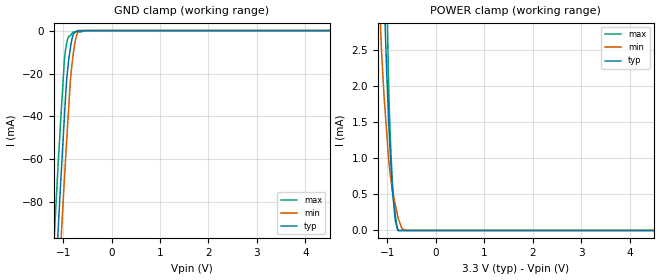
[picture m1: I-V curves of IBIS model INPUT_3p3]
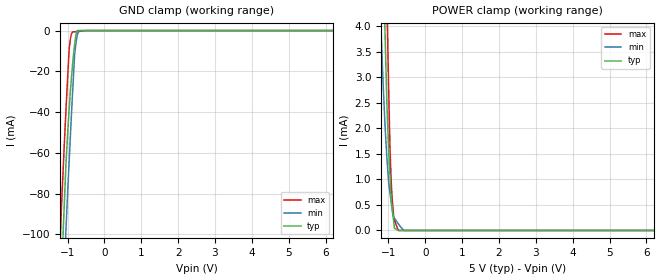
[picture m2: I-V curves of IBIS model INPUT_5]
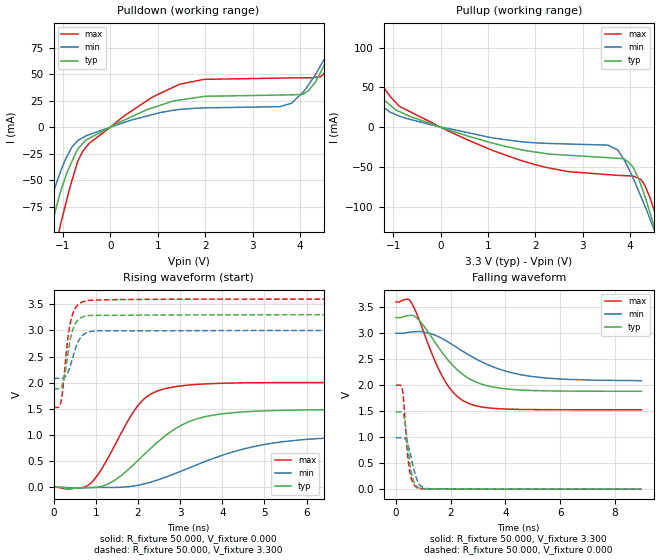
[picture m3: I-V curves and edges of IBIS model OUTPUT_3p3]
|Texas Instruments Incorporated
|14-Bit, Quad Channel, Serial Interface, Multiplying Digital-to-Analog Converter
| Marketing part#   Digital Voltage Range   Package-type   #pins
| DAC8803IDBR   2.7V to 5.5V   SSOP   28
| DAC8803IDBRG4   2.7V to 5.5V   SSOP   28
| DAC8803IDBT   2.7V to 5.5V   SSOP   28
| DAC8803IDBTG4   2.7V to 5.5V   SSOP   28
[IBIS Ver]   3.2
[File name]   dac8803.ibs
|SIMDE Ver   V2.0 - 201002 - RHL4 - Build 372
[Date]   08/20/2010
[File Rev]   1.1
[Source]
| Texas Instruments Incorporated.
| Analog eLab Design Center, HPA
| 12500 TI Blvd
| Dallas, TX -75243
| e-Mail: elab_scm_ibis@list.ti.com
| Model generated from simulations in TISPICE
[Notes]   Revision_History:
|   Rev 1.0: 08/02/2010
|   - Initial version of the model
|   - Model names with a trailing _3p3 contains the model for
|   3V [3 - 3.3 - 3.6]. Model names with trailing _5 contains
|   the model for 5V [4.5 - 5.0 - 5.5] operation.
|   - Model generated from simulations in TISPICE
|   - Model matched to SPICE simulation
|   - While calculating R_pkg, L_pkg and C_pkg ignored values
|   corresponding to power and ground pins
|   - Added package details beside [Package]
|   - C_comp although listed in numerical order of value are
|   obtained from varying PVT conditions. For PVT conditions
|   for each specific value refer the buffer description under
|   respective [Model]. IBIS model user is responsible for using
|   appropriate C_comp to simulate for Signal Integrity.
|   Rev 1.1: 08/20/2010
|   - Re-released after removing INPUT_EN buffers and using INPUT
|   instead
|   - Updated all analog pins as TERM
[Disclaimer]
| This model is designed as an aid for customers of Texas Instruments.
| TI and its licensors and suppliers make no warranties, either expressed
| or implied, with respect to this  model, including the warranties of
| merchantability or fitness for a particular purpose. The model is
| provided solely on an "as is" basis. The entire risk as to its quality
| and performance is with the customer.
[Copyright]
| (C) Copyright 2010 Texas Instruments Incorporated. All rights reserved.
|   DAC8803
[Component]   DAC8803
[Manufacturer]  TI
[Package]  | 28 SSOP - DB package
| variable   typ   min   max
R_pkg   0.03644   0.00363   0.05238
L_pkg   3.09853nH   1.17548nH   4.86282nH
C_pkg   0.73875pF   0.35147pF   1.22787pF
|-------------------------PIN------------------------------------------------
[Pin]  signal_name model_name   R_pin   L_pin   C_pin
1   AGNDA   GND   0.03184   5.81591nH   1.29735pF
2   IOUTA   TERM   0.04659   4.86134nH   1.22696pF
3   VREFA   TERM   0.02815   4.00710nH   1.00527pF
4   RFBA   TERM   0.03031   2.81959nH   0.71201pF
5   MSB   INPUT   0.05211   2.64328nH   0.50891pF
6   _RS   INPUT   0.04857   2.33897nH   0.44307pF
7   VDD   POWER   0.02476   2.03620nH   0.46247pF
8   _CS   INPUT   0.04562   2.25151nH   0.43554pF
9   CLK   INPUT   0.04863   2.34561nH   0.44303pF
10   SDI   INPUT   0.05238   2.65862nH   0.51001pF
11   RFBB   TERM   0.03030   2.82161nH   0.71298pF
12   VREFB   TERM   0.02744   3.75266nH   0.95519pF
13   IOUTB   TERM   0.04608   4.68935nH   1.17882pF
14   AGNDB   GND   0.03363   6.46641nH   1.45119pF
15   AGNDC   GND   0.03286   6.18883nH   1.39946pF
16   IOUTC   TERM   0.04625   4.74353nH   1.19893pF
17   VREFC   TERM   0.02759   3.80912nH   0.95675pF
18   RFBC   TERM   0.03017   2.73838nH   0.68849pF
19   NC   NC   0.00363   1.17548nH   0.37105pF
20   SDO   OUTPUT   0.04717   2.29948nH   0.43486pF
21   _LDAC   INPUT   0.04546   2.24617nH   0.43309pF
22   AGNDF   GND   0.04609   2.26472nH   0.43205pF
23   VSS   NC   0.00371   1.17578nH   0.35147pF
24   DGND   GND   0.02988   2.49325nH   0.54126pF
25   RFBD   TERM   0.03031   2.82053nH   0.71469pF
26   VREFD   TERM   0.02815   4.00814nH   1.00483pF
27   IOUTD   TERM   0.04661   4.86282nH   1.22787pF
28   AGNDD   GND   0.03187   5.81892nH   1.29817pF
|   Model Selectors
[Model Selector]  INPUT
INPUT_3p3  3V digital input
INPUT_5   5V digital input
|NOTES   Model INPUT split into two Models INPUT_3p3 and INPUT_5
|   to accomodate vast voltage range of 2.7V - 5.5V
|   INPUT_3p3 operates in voltage range of 3.0 - 3.3 - 3.6
|   INPUT_5 operates in voltage range of 4.5 - 5.0 - 5.5
|   The max pin frequency for Model INPUT is 20MHz
|   This is referenced with datasheet
[Model Selector]  OUTPUT
OUTPUT_3p3   3V digital output
OUTPUT_5   5V digital output
|NOTES   Model OUTPUT split into two Models OUTPUT_3p3 and OUTPUT_5
|   to accomodate vast voltage range of 2.7V - 5.5V
|   OUTPUT_3p3 operates in voltage range of 3.0 - 3.3 - 3.6
|   OUTPUT_5 operates in voltage range of 4.5 - 5.0 - 5.5
|   The max pin frequency for Model OUTPUT is 12.5MHz
|   This is referenced with datasheet
[Model selector] TERM
TERM_3p3  3.3V nominal termination
TERM_5   5.0V nominal termination
|   Termination - TERM_3p3
[Model] TERM_3p3
Model_type Terminator
C_comp   1.0e-20F  1.0e-20F  1.0e-20F
| variable   typ   min   max
[Voltage Range]   3.30000v  3.00000V  3.60000V
[POWER Clamp Reference]  3.30000v  3.00000V  3.60000V
[GND Clamp Reference]   0.00000V  0.00000V  0.00000V
|Ambient Temperature   25   85   -40
|Junction Temperature
[Temperature Range]   25   85   -40
|   Termination - TERM_5
[Model] TERM_5
Model_type Terminator
C_comp   1.0e-20F  1.0e-20F  1.0e-20F
| variable   typ   min   max
[Voltage Range]   5.00000V  4.50000V  5.50000V
[POWER Clamp Reference]  5.00000V  4.50000V  5.50000V
[GND Clamp Reference]   0.00000V  0.00000V  0.00000V
|Ambient Temperature   25   85   -40
|Junction Temperature
[Temperature Range]   25   85   -40
| Models and submodels in the file (6): INPUT_3p3 (Input), INPUT_5 (Input), OUTPUT_3p3 (Output), OUTPUT_5 (Output), TERM_3p3 (Terminator), TERM_5 (Terminator)
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|   Input INPUT 3 Model
[Model] INPUT_3p3
Model_type Input
| Signals   MSB(5), _RS(6), _LDAC(21)
Vinl = 0.6
Vinh = 2.1
|   typ   min   max
|   (nom PVT)   (Fast PVT)   (slow PVT)
C_comp   7.483e-13   7.448e-13   7.667e-13
| Where   nom PVT is  Nominal Process, 3.3V, 25C
|   Fast PVT is Strong Process, 3.6V, -40C
|   Slow PVT is Weak Process, 3.0V, 85C
[Voltage Range]   3.3   3   3.6
|Ambient Temperature   25   85   -40
|Junction Temperature
[Temperature Range]   25   85   -40
[Power Clamp Reference]   3.3   3   3.6
[GND Clamp Reference]   0   0   0
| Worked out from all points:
|   GND clamp passes 1 mA (typ) near -0.77 V on its own axis
|   POWER clamp passes 1 mA (typ) near -0.93 V on its own axis
[GND Clamp]
|   Voltage   I(typ)   I(min)   I(max)
-3.3V     -1.166A    -1.193A    -1.14A
-1.224V   -146.7mA   -178.5mA   -114.6mA
-1.172V   -123mA     -154.8mA   -90.55mA
-1.129V   -103mA     -135mA     -72.36mA
-1.1V     -91.13mA   -122.3mA   -60.64mA
-1.036V   -64.11mA   -93.89mA   -35.55mA
-970.8mV  -38.4mA    -67.62mA   -12.36mA
-884.4mV  -13.28mA   -34.85mA   -2.608mA
-794.4mV  -2.063mA   -11.11mA   -710.2uA
-723mV    -267.5uA   -2.257mA   -615.5uA
-640.2mV  0A         0A         -594uA
6.6V      0A         0A         0A
[POWER Clamp]
|   Voltage   I(typ)   I(min)   I(max)
-3.3V     92.94mA    75.28mA    116.7mA
-1.172V   6.217mA    3.285mA    9.654mA
-1.132V   4.864mA    2.662mA    7.996mA
-1.068V   3.289mA    1.855mA    5.414mA
-1.013V   2.168mA    1.341mA    3.379mA
-978mV    1.604mA    1.013mA    2.134mA
-938.4mV  1.049mA    765.5uA    1.257mA
-902.4mV  629uA      574.6uA    731.3uA
-834.9mV  130.7uA    352.7uA    207.6uA
-780mV    0A         177.8uA    0A
-603mV    0A         0A         0A
6.6V      0A         0A         0A
|   Input INPUT 5 Model
[Model] INPUT_5
Model_type Input
| Signals   MSB(5), _RS(6), _LDAC(21)
Vinl = 0.8
Vinh = 2.4
|   typ   min   max
|   (nom PVT)   (Fast PVT)   (slow PVT)
C_comp   7.000e-13   6.968e-13   7.186e-13
| Where   nom PVT is  Nominal Process, 5.0V, 25C
|   Fast PVT is Strong Process, 5.5V, -40C
|   Slow PVT is Weak Process, 4.5V, 85C
[Voltage Range]   5   4.5   5.5
|Ambient Temperature   25   85   -40
|Junction Temperature
[Temperature Range]   25   85   -40
[Power Clamp Reference]   5   4.5   5.5
[GND Clamp Reference]   0   0   0
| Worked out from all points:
|   GND clamp passes 1 mA (typ) near -0.76 V on its own axis
|   POWER clamp passes 1 mA (typ) near -0.95 V on its own axis
[GND Clamp]
|   Voltage   I(typ)   I(min)   I(max)
-5V       -2.016A    -2.04A     -1.994A
-1.198V   -134.6mA   -166.3mA   -102.4mA
-1.145V   -110.8mA   -142.4mA   -78.84mA
-1.089V   -86.12mA   -117.2mA   -56.59mA
-1.045V   -66.57mA   -98.85mA   -39.96mA
-952mV    -37.7mA    -62.86mA   -8.495mA
-864mV    -16.96mA   -30.99mA   -628.8uA
-806mV    -6.872mA   -11.51mA   -603.2uA
-774.5mV  -2.572mA   -6.593mA   -594.5uA
-702.5mV  0A         -440.8uA   -484.3uA
-635mV    0A         0A         -315.3uA
10V       0A         0A         0A
[POWER Clamp]
|   Voltage   I(typ)   I(min)   I(max)
-5V       164.7mA    136.8mA    204.1mA
-1.234V   8.352mA    4.605mA    12.5mA
-1.167V   6.176mA    3.308mA    9.386mA
-1.095V   3.971mA    2.115mA    6.474mA
-1.035V   2.356mA    1.36mA     4.24mA
-1.024V   2.143mA    1.244mA    3.831mA
-957.5mV  1.079mA    740.3uA    1.621mA
-908mV    521.2uA    468.4uA    734.6uA
-835mV    42.37uA    238.8uA    203.6uA
-732mV    0A         131.7uA    0A
-581mV    0A         0A         0A
10V       0A         0A         0A
|   Output OUTPUT 3 Model
[Model] OUTPUT_3p3
Model_type Output
|Signal SDO(20) pin
Polarity   Non-Inverting
Enable   Active-Low
Vmeas = 1.65
Vref = 1.65
Cref = 15pF
Rref = 50
|   typ   min   max
|   (nom PVT)   (Fast PVT)   (slow PVT)
|Average
C_comp   4.561e-12   4.188e-12   4.582e-12
|ON state : BUFFER OUTPUT TURNED HIGH
|C_comp   4.045e-12   3.857e-12   4.639e-12
|OFF state: BUFFER in HIGH IMPEDANCE for IOs and 3-state,
|This is BUFFER in LOW state for OUTPUT only type
|C_comp   4.524e-12   4.331e-12   5.266e-12
| Where   nom PVT is  Nominal Process, 3.3V, 25C
|   Fast PVT is Strong Process, 3.6V, -40C
|   Slow PVT is Weak Process, 3.0V, 85C
[Voltage Range]   3.3   3   3.6
|Ambient Temperature   25   85   -40
|Junction Temperature
[Temperature Range]   25   85   -40
[Pullup Reference]   3.3   3   3.6
[Pulldown Reference]   0   0   0
[Power Clamp Reference]   3.3   3   3.6
[GND Clamp Reference]   0   0   0
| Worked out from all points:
|   slope of the pulldown table from 0 to 0.495 V, typ, clamps not added: 45.7 ohm
|   slope of the pullup table from 0 to 0.495 V, typ, clamps not added: 50.9 ohm
|   falling waveform, R_fixture 50.000, V_fixture 3.300: 20-80 % time 1.37ns typ, 2.07ns min, 1.07ns max; typ from 3.3 V to 1.88 V
|   rising waveform, R_fixture 50.000, V_fixture 0.000: 20-80 % time 1.33ns typ, 2.13ns min, 864ps max; typ from 0 V to 1.49 V
|   rising waveform, R_fixture 50.000, V_fixture 3.300: 20-80 % time 189ps typ, 231ps min, 180ps max; typ from 1.88 V to 3.3 V
|   falling waveform, R_fixture 50.000, V_fixture 0.000: 20-80 % time 217ps typ, 287ps min, 191ps max; typ from 1.49 V to 0 V
[Pulldown]
|   Voltage   I(typ)   I(min)   I(max)
-3.3V     -563.8mA   -410.1mA   -812.5mA
-1.576V   -164.7mA   -116.8mA   -237.6mA
-1.316V   -109.3mA   -77.56mA   -156.7mA
-1.122V   -72.09mA   -50.69mA   -106.5mA
-719.4mV  -23.2mA    -14.26mA   -36.79mA
-448.8mV  -10.6mA    -7.092mA   -15.39mA
1.466V    25.59mA    16.71mA    40.53mA
3.822V    30.47mA    22.51mA    46.48mA
4.316V    41.7mA     48.63mA    46.94mA
4.724V    79.23mA    81.02mA    69.4mA
5.67V     172.5mA    157.1mA    190.6mA
6.6V      257.3mA    225.7mA    301.3mA
[Pullup]
|   Voltage   I(typ)   I(min)   I(max)
-3.3V     224.9mA    184mA      283.1mA
-2.581V   161.9mA    130.6mA    206mA
-1.565V   64.84mA    50.24mA    83.44mA
-1.23V    37.53mA    26.18mA    52.54mA
-870mV    19.61mA    13.9mA     26.2mA
1.69V     -28.33mA   -18.3mA    -41.78mA
3.738V    -39.18mA   -28.47mA   -60.64mA
4.069V    -51.04mA   -64.76mA   -61.79mA
4.3V      -84.61mA   -97.27mA   -71.98mA
4.501V    -123.5mA   -127.9mA   -102.9mA
4.635V    -151.5mA   -148.8mA   -131.9mA
6.6V      -606.2mA   -488.2mA   -776.3mA
[Ramp]
R_load = 50
|   typ   min   max
dV/dt_r   0.892569/1.32425e-09   0.589705/2.12777e-09   1.20285/8.6344e-10
dV/dt_f   0.861496/1.37049e-09   0.547821/2.07275e-09   1.24372/1.0702e-09
[Falling Waveform]
R_fixture = 50.000
V_fixture = 3.300
V_fixture_min = 3.000
V_fixture_max = 3.600
C_fixture = 0.000
|  time   V(typ)   V(min)   V(max)
0s        3.3V       3V         3.6V
525ps     3.342V     3.022V     3.616V
900ps     3.217V     3.032V     3.18V
1.4ns     2.847V     2.968V     2.496V
1.75ns    2.586V     2.879V     2.117V
2.175ns   2.329V     2.742V     1.816V
2.65ns    2.134V     2.587V     1.65V
3.55ns    1.964V     2.352V     1.555V
4.9ns     1.899V     2.173V     1.532V
8.975ns   1.883V     2.087V     1.527V
[Rising Waveform]
R_fixture = 50.000
V_fixture = 0.000
V_fixture_min = 0.000
V_fixture_max = 0.000
C_fixture = 0.000
|  time   V(typ)   V(min)   V(max)
0s        1.175nV    1.317nV    988.8pV
350ps     -24.78mV   -8.949mV   -35.56mV
875ps     -5.93mV    -5.321mV   72.33mV
1.35ns    86.77mV    -3.196mV   646.5mV
1.975ns   490.9mV    34.13mV    1.537V
2.25ns    703.5mV    85.93mV    1.756V
2.625ns   969.4mV    183.6mV    1.883V
3.6ns     1.352V     494.7mV    1.977V
5.175ns   1.466V     841.8mV    2.001V
8.975ns   1.488V     982.8mV    2.005V
[Rising Waveform]
R_fixture = 50.000
V_fixture = 3.300
V_fixture_min = 3.000
V_fixture_max = 3.600
C_fixture = 0.000
|  time   V(typ)   V(min)   V(max)
0s        1.883V     2.084V     1.527V
125ps     1.882V     2.084V     1.534V
175ps     1.903V     2.082V     1.626V
250ps     2.085V     2.096V     2.11V
325ps     2.465V     2.172V     2.751V
425ps     2.929V     2.394V     3.237V
575ps     3.198V     2.77V      3.488V
725ps     3.269V     2.929V     3.557V
1.1ns     3.289V     2.994V     3.583V
8.975ns   3.3V       3V         3.6V
[Falling Waveform]
R_fixture = 50.000
V_fixture = 0.000
V_fixture_min = 0.000
V_fixture_max = 0.000
C_fixture = 0.000
|  time   V(typ)   V(min)   V(max)
0s        1.486V     989mV      2.001V
225ps     1.476V     990.1mV    1.933V
275ps     1.428V     987.9mV    1.728V
325ps     1.303V     974.4mV    1.375V
425ps     868.7mV    871.7mV    661mV
500ps     532.5mV    728.2mV    349.6mV
625ps     187.4mV    443mV      118.6mV
800ps     39.54mV    143.4mV    21.16mV
1.25ns    6.306mV    7.231mV    7.266mV
8.975ns   220.9uV    317.2uV    79.42uV
